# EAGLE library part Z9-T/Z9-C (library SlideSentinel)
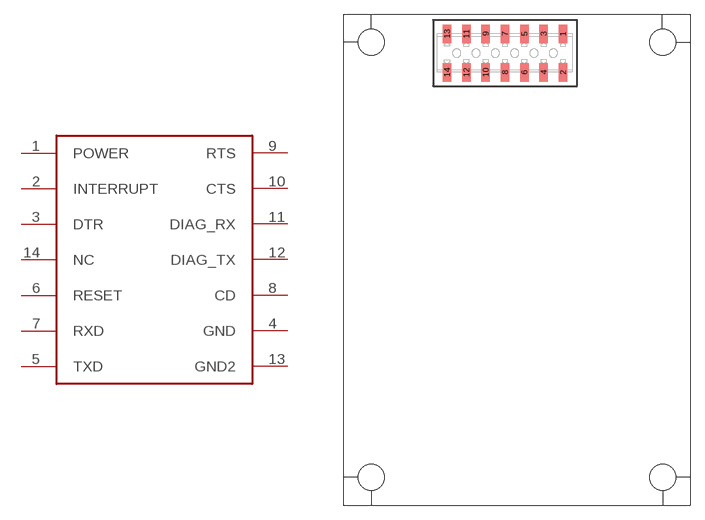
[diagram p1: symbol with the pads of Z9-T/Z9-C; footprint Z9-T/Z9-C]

Designator prefix -

## Z9-T/Z9-C  [Z9-T/Z9-C]
1  POWER
2  INTERRUPT
3  DTR
4  GND
5  TXD
6  RESET
7  RXD
8  CD
9  RTS
10  CTS
11  DIAG_RX
12  DIAG_TX
13  GND2
14  NC

## Footprint Z9-T/Z9-C (pad centres in mm)
translated Allegro footprint
smd 0.89 x 1.91: 1 6,2; 2 6,-2; 3 4,2; 4 4,-2; 5 2,2; 6 2,-2; 7 0,2; 8 0,-2; 9 -2,2; 10 -2,-2; 11 -4,2; 12 -4,-2; 13 -6,2; 14 -6,-2
hole 2.7 at -13.832,1.122
hole 2.7 at -13.832,-43.922
hole 2.7 at 16.302,-43.912
hole 2.7 at 16.302,1.122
